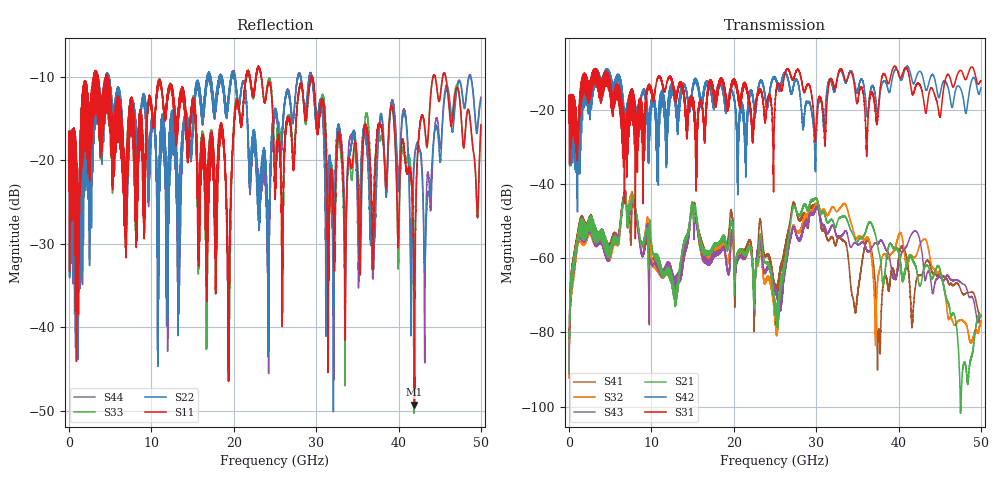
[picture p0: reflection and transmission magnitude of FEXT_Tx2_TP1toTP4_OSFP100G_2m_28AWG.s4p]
! Touchstone data
! Created: 27-Feb-2019 by IdEM 12 (12.1.0)
! COMMENTS
!  Created Wed Feb 27 12:03:36 2019
!  64 Port Network Data from SP1.SP block
!  freq  magS1_1  angS1_1  magS1_2  angS1_2  magS1_3  angS1_3  magS1_4  angS1_4
!  magS1_5  angS1_5  magS1_6  angS1_6  magS1_7  angS1_7  magS1_8  angS1_8
!  magS1_9  angS1_9  magS1_10  angS1_10  magS1_11  angS1_11  magS1_12  angS1_12
!  magS1_13  angS1_13  magS1_14  angS1_14  magS1_15  angS1_15  magS1_16  angS1_16
!  magS1_17  angS1_17  magS1_18  angS1_18  magS1_19  angS1_19  magS1_20  angS1_20
!  magS1_21  angS1_21  magS1_22  angS1_22  magS1_23  angS1_23  magS1_24  angS1_24
!  magS1_25  angS1_25  magS1_26  angS1_26  magS1_27  angS1_27  magS1_28  angS1_28
!  magS1_29  angS1_29  magS1_30  angS1_30  magS1_31  angS1_31  magS1_32  angS1_32
!  magS1_33  angS1_33  magS1_34  angS1_34  magS1_35  angS1_35  magS1_36  angS1_36
!  magS1_37  angS1_37  magS1_38  angS1_38  magS1_39  angS1_39  magS1_40  angS1_40
!  magS1_41  angS1_41  magS1_42  angS1_42  magS1_43  angS1_43  magS1_44  angS1_44
!  magS1_45  angS1_45  magS1_46  angS1_46  magS1_47  angS1_47  magS1_48  angS1_48
!  magS1_49  angS1_49  magS1_50  angS1_50  magS1_51  angS1_51  magS1_52  angS1_52
!  magS1_53  angS1_53  magS1_54  angS1_54  magS1_55  angS1_55  magS1_56  angS1_56
!  magS1_57  angS1_57  magS1_58  angS1_58  magS1_59  angS1_59  magS1_60  angS1_60
!  magS1_61  angS1_61  magS1_62  angS1_62  magS1_63  angS1_63  magS1_64  angS1_64
!  magS2_1  angS2_1  magS2_2  angS2_2  magS2_3  angS2_3  magS2_4  angS2_4
!  magS2_5  angS2_5  magS2_6  angS2_6  magS2_7  angS2_7  magS2_8  angS2_8
!  magS2_9  angS2_9  magS2_10  angS2_10  magS2_11  angS2_11  magS2_12  angS2_12
!  magS2_13  angS2_13  magS2_14  angS2_14  magS2_15  angS2_15  magS2_16  angS2_16
!  magS2_17  angS2_17  magS2_18  angS2_18  magS2_19  angS2_19  magS2_20  angS2_20
!  magS2_21  angS2_21  magS2_22  angS2_22  magS2_23  angS2_23  magS2_24  angS2_24
!  magS2_25  angS2_25  magS2_26  angS2_26  magS2_27  angS2_27  magS2_28  angS2_28
!  magS2_29  angS2_29  magS2_30  angS2_30  magS2_31  angS2_31  magS2_32  angS2_32
!  magS2_33  angS2_33  magS2_34  angS2_34  magS2_35  angS2_35  magS2_36  angS2_36
!  magS2_37  angS2_37  magS2_38  angS2_38  magS2_39  angS2_39  magS2_40  angS2_40
!  magS2_41  angS2_41  magS2_42  angS2_42  magS2_43  angS2_43  magS2_44  angS2_44
!  magS2_45  angS2_45  magS2_46  angS2_46  magS2_47  angS2_47  magS2_48  angS2_48
!  magS2_49  angS2_49  magS2_50  angS2_50  magS2_51  angS2_51  magS2_52  angS2_52
!  magS2_53  angS2_53  magS2_54  angS2_54  magS2_55  angS2_55  magS2_56  angS2_56
!  magS2_57  angS2_57  magS2_58  angS2_58  magS2_59  angS2_59  magS2_60  angS2_60
!  magS2_61  angS2_61  magS2_62  angS2_62  magS2_63  angS2_63  magS2_64  angS2_64
!  magS3_1  angS3_1  magS3_2  angS3_2  magS3_3  angS3_3  magS3_4  angS3_4
!  magS3_5  angS3_5  magS3_6  angS3_6  magS3_7  angS3_7  magS3_8  angS3_8
!  magS3_9  angS3_9  magS3_10  angS3_10  magS3_11  angS3_11  magS3_12  angS3_12
!  magS3_13  angS3_13  magS3_14  angS3_14  magS3_15  angS3_15  magS3_16  angS3_16
!  magS3_17  angS3_17  magS3_18  angS3_18  magS3_19  angS3_19  magS3_20  angS3_20
!  magS3_21  angS3_21  magS3_22  angS3_22  magS3_23  angS3_23  magS3_24  angS3_24
!  magS3_25  angS3_25  magS3_26  angS3_26  magS3_27  angS3_27  magS3_28  angS3_28
!  magS3_29  angS3_29  magS3_30  angS3_30  magS3_31  angS3_31  magS3_32  angS3_32
!  magS3_33  angS3_33  magS3_34  angS3_34  magS3_35  angS3_35  magS3_36  angS3_36
!  magS3_37  angS3_37  magS3_38  angS3_38  magS3_39  angS3_39  magS3_40  angS3_40
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# Hz S MA R 50
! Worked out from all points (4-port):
!   5000 points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, 10 MHz to 50 GHz, reference 50 ohm
!   strongest paths, dB at 10 MHz, 12.51 GHz, 25.01 GHz, 37.51 GHz, 50 GHz:
!     S31: -18.0, -12.2, -18.3, -20.7, -12.2
!     S42: -18.0, -13.8, -11.3, -20.6, -14.1
!     S21: -90.6, -65.5, -73.8, -57.1, -75.8
!     S43: -91.1, -64.5, -68.3, -56.2, -75.4
!     S32: -92.3, -64.2, -76.5, -65.1, -77.0
!     S41: -89.4, -65.8, -67.8, -83.1, -75.6
!   lowest |S11| = -49.3 dB at 41.94 GHz (marker M1), VSWR 1.01, Z = 49.7 - j0.0423 ohm
!   |S11| at or under -10 dB: 4.661 GHz to 21.47 GHz (16.81 GHz wide, 129 % of centre); 23.35 GHz to 29.41 GHz (6.055 GHz wide, 23 % of centre); 29.53 GHz to 44.21 GHz (14.68 GHz wide, 39.8 % of centre)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
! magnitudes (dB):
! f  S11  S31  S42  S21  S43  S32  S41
! 10 MHz  -17.7  -18.0  -18.0  -90.6  -91.1  -92.3  -89.4
! 6.7 GHz  -27.9  -25.6  -22.7  -43.4  -42.7  -43.4  -42.6
! 25.19 GHz  -19.8  -13.9  -12.0  -78.1  -68.8  -77.2  -69.8
! 29.78 GHz  -11.7  -24.3  -28.7  -44.3  -47.8  -46.8  -46.2
! 37.6 GHz  -15.9  -18.6  -19.3  -58.2  -55.8  -64.1  -79.5
! 41.94 GHz  -49.3  -14.8  -12.7  -61.4  -52.7  -59.8  -69.9
! 50 GHz  -15.7  -12.2  -14.1  -75.8  -75.4  -77.0  -75.6
